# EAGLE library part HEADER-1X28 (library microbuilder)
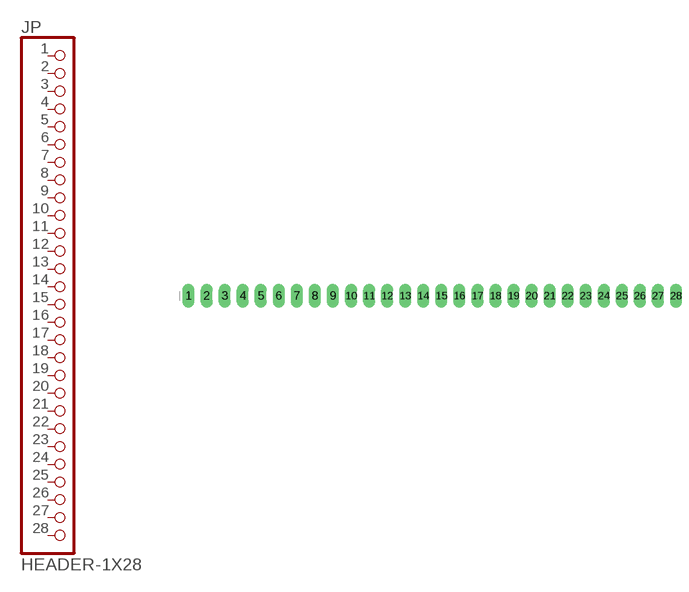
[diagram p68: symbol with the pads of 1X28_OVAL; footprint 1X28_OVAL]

Designator prefix JP

## HEADER-1X28  [1X28_OVAL]
1  1  pas
2  2  pas
3  3  pas
4  4  pas
5  5  pas
6  6  pas
7  7  pas
8  8  pas
9  9  pas
10  10  pas
11  11  pas
12  12  pas
13  13  pas
14  14  pas
15  15  pas
16  16  pas
17  17  pas
18  18  pas
19  19  pas
20  20  pas
21  21  pas
22  22  pas
23  23  pas
24  24  pas
25  25  pas
26  26  pas
27  27  pas
28  28  pas

## Footprint 1X28_OVAL (pad centres in mm)
drill 1 pad 1.676 long: 1 -34.29,0; 2 -31.75,0; 3 -29.21,0; 4 -26.67,0; 5 -24.13,0; 6 -21.59,0; 7 -19.05,0; 8 -16.51,0; 9 -13.97,0; 10 -11.43,0; 11 -8.89,0; 12 -6.35,0; 13 -3.81,0; 14 -1.27,0; 15 1.27,0; 16 3.81,0; 17 6.35,0; 18 8.89,0; 19 11.43,0; 20 13.97,0; 21 16.51,0; 22 19.05,0; 23 21.59,0; 24 24.13,0; 25 26.67,0; 26 29.21,0; 27 31.75,0; 28 34.29,0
